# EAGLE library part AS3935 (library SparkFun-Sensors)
AS3935 Franklin Lightning Sensor The AS3935 is a programmable fully integrated Lightning Sensor IC that detects the presence and approach of potentially hazardous lightning activity in the vicinity and provides an estimation on the distance to the head of the storm. The embedded lightning algorithm checks the incoming signal pattern to reject the potential man-made disturbers.The AS3935 can also provide information on the noise level and inform the external unit (e.g. microcontroller) in case of high noise conditions, with the noise floor generator and noise floor evaluation blocks.
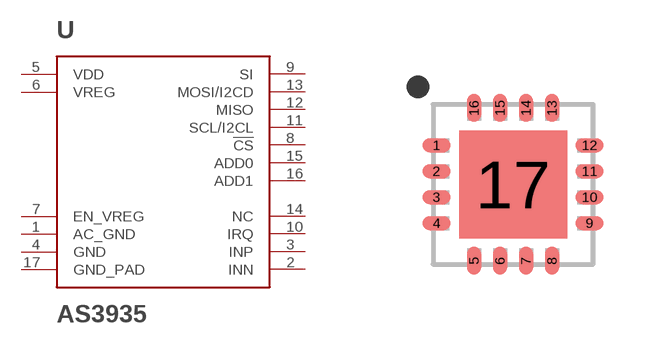
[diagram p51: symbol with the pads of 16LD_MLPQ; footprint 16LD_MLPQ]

Designator prefix U

## AS3935QFN (PROD_ID: IC-11333; VALUE: AS3935)  [16LD_MLPQ]
1  AC_GND  pwr
2  INN
3  INP
4  GND  pwr
5  VDD  pwr
6  VREG  pwr
7  EN_VREG
8  !CS  in
9  SI  in
10  IRQ
11  SCL/I2CL  in
12  MISO  out
13  MOSI/I2CD  in
14  NC  nc
15  ADD0  in
16  ADD1  in
17  GND_PAD  pwr

## Footprint 16LD_MLPQ (pad centres in mm)
MLPQ-16 Dimensions 4mm x 4mm x .75mm 16 Pin Exposed ground pad underneath
smd 0.7 x 0.35: 1 -1.919,0.968; 2 -1.919,0.318; 3 -1.919,-0.332; 4 -1.919,-0.982; 9 1.908,-0.982; 10 1.908,-0.332; 11 1.908,0.318; 12 1.908,0.968
smd 0.35 x 0.7: 5 -0.982,-1.917; 6 -0.332,-1.917; 7 0.318,-1.917; 8 0.968,-1.917; 13 0.968,1.907; 14 0.318,1.907; 15 -0.332,1.907; 16 -0.982,1.907
smd 2.7 x 2.7: 17 -0.007,-0.007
